ORGANIZATION_BLOCK OB 100
BEGIN
	// Check DB/DI register assignments
	__ASSERT==	__DBR 1,	0
	__ASSERT==	__DBR 2,	0
	AUF		DB 1
	__ASSERT==	__DBR 1,	1
	__ASSERT==	__DBR 2,	0
	AUF		DB 2
	__ASSERT==	__DBR 1,	2
	__ASSERT==	__DBR 2,	0
	AUF		DI 1
	__ASSERT==	__DBR 1,	2
	__ASSERT==	__DBR 2,	1
	AUF		DI 2
	__ASSERT==	__DBR 1,	2
	__ASSERT==	__DBR 2,	2


	// Check initial DB 1 values
	AUF		DB 1
	L		DBW 0
	__ASSERT==	__ACCU 1,	1337
	L		DBD 2
	__ASSERT==	__ACCU 1,	DW#16#DEADBEEF
	L		DBW 6
	__ASSERT==	__ACCU 1,	W#16#0102
	L		DBB 8
	__ASSERT==	__ACCU 1,	3
	L		DBB 9
	__ASSERT==	__ACCU 1,	0
	L		DBW 10
	__ASSERT==	__ACCU 1,	42

	// Check initial DB 2 values
	AUF		DB 2
	L		DBW 0
	__ASSERT==	__ACCU 1,	123
	L		DBW 2
	__ASSERT==	__ACCU 1,	456
	L		DBB 4
	__ASSERT==	__ACCU 1,	1
	L		DBB 5
	__ASSERT==	__ACCU 1,	0
	L		DBD 6
	__ASSERT==	__ACCU 1,	DW#16#77777777


	// Check direct DB fetch
	AUF		DB 2
	__ASSERT==	__DBR 1,	2
	L		DB1.DBW 0
	__ASSERT==	__DBR 1,	1
	__ASSERT==	__ACCU 1,	1337
	L		DB1.DBD 2
	__ASSERT==	__DBR 1,	1
	__ASSERT==	__ACCU 1,	DW#16#DEADBEEF
	L		DB1.DBW 6
	__ASSERT==	__DBR 1,	1
	__ASSERT==	__ACCU 1,	W#16#0102
	L		DB1.DBB 8
	__ASSERT==	__DBR 1,	1
	__ASSERT==	__ACCU 1,	3
	L		DB1.DBB 9
	__ASSERT==	__DBR 1,	1
	__ASSERT==	__ACCU 1,	0
	L		DB1.DBW 10
	__ASSERT==	__DBR 1,	1
	__ASSERT==	__ACCU 1,	42
	AUF		DB 1
	__ASSERT==	__DBR 1,	1
	L		DB2.DBW 0
	__ASSERT==	__DBR 1,	2
	__ASSERT==	__ACCU 1,	123


	SET
	=		M 0.0
END_ORGANIZATION_BLOCK



ORGANIZATION_BLOCK OB 1
BEGIN
	// OB 100 execution sanity check
	__ASSERT==	M 0.0,		1

	// Modify the DB 1
	AUF		DB 1
	L		9876
	T		DBW 6
	L		5432
	T		DBW 10
	CLR
	=		DBX 8.0
	SET
	=		DBX 8.2

	// Check the DB 1 values
	L		DBW 0
	__ASSERT==	__ACCU 1,	1337
	L		DBD 2
	__ASSERT==	__ACCU 1,	DW#16#DEADBEEF
	L		DBW 6
	__ASSERT==	__ACCU 1,	9876
	L		DBB 8
	__ASSERT==	__ACCU 1,	6
	L		DBB 9
	__ASSERT==	__ACCU 1,	0
	L		DBW 10
	__ASSERT==	__ACCU 1,	5432


	// Check direct DB store
	AUF		DB 2	// DB 2 on purpose
	L		2244
	T		DB1.DBW 6
	L		L#1008901
	T		DB1.DBD 2
	SET
	=		DB1.DBX 8.0
	L		42
	T		DB1.DBB 9

	L		DB1.DBW 6
	__ASSERT==	__ACCU 1,	2244
	L		DB1.DBD 2
	__ASSERT==	__ACCU 1,	L#1008901
	U		DB1.DBX 8.0
	__ASSERT==	__STW VKE,	1
	L		DB1.DBB 9
	__ASSERT==	__ACCU 1,	42


	// FB 1 call test
	CLR
	=		M 18.0
	CALL		FB 1, DB 2 (
		INPUT_VAR	:= 8877,
		OUTPUT_VAR	:= LW 16,
		INOUT_VAR	:= M 18.0
	)
	__ASSERT==	LW 16,		4433
	__ASSERT==	M 18.0,		1


	// FC 1 call test
	L		1616
	T		LW 16
	L		2020
	T		MW 20
	CALL		FC 1 (
		INPUT_WORD	:= LW 16,
		INPUT_FC	:= FC 2,
		INPUT_FB	:= FB 1,
		INPUT_DB	:= DB 1,
		OUTPUT_BOOL0	:= M 18.0,
		OUTPUT_BOOL1	:= M 18.1,
		INOUT_INT	:= MW 20
	)
	__ASSERT==	M 18.0,		1
	__ASSERT==	M 18.1,		0


	// Check DB/DI register assignments around FC/FB calls
	AUF		DB 12
	AUF		DI 13
	__ASSERT==	__DBR 1,	12
	__ASSERT==	__DBR 2,	13
	CALL		FC 10
	__ASSERT==	__DBR 1,	12
	__ASSERT==	__DBR 2,	13
	CALL		FB 11, DB 11
	__ASSERT==	__DBR 1,	11
	__ASSERT==	__DBR 2,	13


	// Check DBNO, DINO, DBLG and DILG operators
	AUF		DB 1
	AUF		DI 2
	L		DBNO
	__ASSERT==	__ACCU 1,	1
	L		DINO
	__ASSERT==	__ACCU 1,	2
	L		DBLG
	__ASSERT==	__ACCU 1,	12
	L		DILG
	__ASSERT==	__ACCU 1,	10


	CALL SFC 46 // STOP CPU
END_ORGANIZATION_BLOCK



FUNCTION FC 1: VOID
	VAR_INPUT
		INPUT_WORD	: WORD
		INPUT_FC	: BLOCK_FC
		INPUT_FB	: BLOCK_FB
		INPUT_DB	: BLOCK_DB
	END_VAR
	VAR_OUTPUT
		OUTPUT_BOOL0	: BOOL
		OUTPUT_BOOL1	: BOOL
	END_VAR
	VAR_IN_OUT
		INOUT_INT	: INT
	END_VAR
	VAR_TEMP
		TEMP0		: INT
		TEMP1		: BOOL
		TEMP2		: INT
	END_VAR
BEGIN
	L		#INPUT_WORD
	__ASSERT==	__ACCU 1,	1616

	L		#INOUT_INT
	__ASSERT==	__ACCU 1,	2020

	SET
	=		#OUTPUT_BOOL0
	CLR
	=		#OUTPUT_BOOL1

	L		4343
	T		#TEMP0
	SET
	=		#TEMP1
	L		6565
	T		#TEMP2
	__ASSERT==	LW 0,	4343
	__ASSERT==	L 2.0,	1
	__ASSERT==	LW 4,	6565


	// Check the passed-in DB
	AUF		#INPUT_DB
	L		DBW 0
	__ASSERT==	__ACCU 1,	1337
END_FUNCTION



FUNCTION_BLOCK FB 1
	VAR_INPUT
		INPUT_VAR	: INT
	END_VAR
	VAR_OUTPUT
		OUTPUT_VAR	: INT
	END_VAR
	VAR_IN_OUT
		INOUT_VAR	: BOOL
	END_VAR
	VAR
		STAT_VAR	: DWORD
	END_VAR
BEGIN
	L		#INPUT_VAR
	__ASSERT==	__ACCU 1,	8877

	L		4433
	T		#OUTPUT_VAR

	U		#INOUT_VAR
	__ASSERT==	__STW VKE,	0
	SET
	=		#INOUT_VAR

	L		#STAT_VAR
	__ASSERT==	__ACCU 1,	DW#16#77777777
END_FUNCTION_BLOCK



FUNCTION FC 10 : VOID
BEGIN
	__ASSERT==	__DBR 1,	12
	__ASSERT==	__DBR 2,	13
	AUF		DB 1
	AUF		DI 2
	__ASSERT==	__DBR 1,	1
	__ASSERT==	__DBR 2,	2
END_FUNCTION



FUNCTION_BLOCK FB 11
BEGIN
	__ASSERT==	__DBR 1,	13
	__ASSERT==	__DBR 2,	11
	AUF		DB 1
	AUF		DI 2
	__ASSERT==	__DBR 1,	1
	__ASSERT==	__DBR 2,	2
END_FUNCTION_BLOCK



DATA_BLOCK DB 1
TITLE = global DB
STRUCT
	VARIABLE0	: INT
	VARIABLE1	: DWORD
	VARIABLE2	: WORD
	VARIABLE3	: BOOL
	VARIABLE4	: BOOL
	VARIABLE5	: BOOL
	VARIABLE6	: INT
END_STRUCT
BEGIN
	VARIABLE0	:= 1337
	VARIABLE1	:= DW#16#DEADBEEF
	VARIABLE2	:= B#(1, 2)
	VARIABLE3	:= True
	VARIABLE4	:= True
	VARIABLE5	:= False
	VARIABLE6	:= 42
END_DATA_BLOCK



DATA_BLOCK DB 2
TITLE = instance DB for FB 1
FB 1
BEGIN
	INPUT_VAR	:= 123
	OUTPUT_VAR	:= 456
	INOUT_VAR	:= True
	STAT_VAR	:= DW#16#77777777
END_DATA_BLOCK



DATA_BLOCK DB 11
TITLE = instance DB for FB 11
FB 11
BEGIN
END_DATA_BLOCK



DATA_BLOCK DB 12
TITLE = global data block 12
STRUCT
	foo		: INT
END_STRUCT
BEGIN
	foo		:= 12
END_DATA_BLOCK



DATA_BLOCK DB 13
TITLE = global data block 13
STRUCT
	bar		: INT
END_STRUCT
BEGIN
	bar		:= 13
END_DATA_BLOCK
